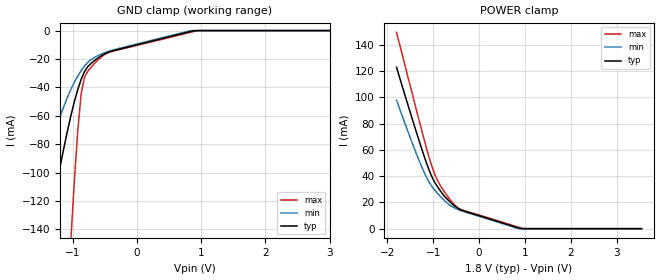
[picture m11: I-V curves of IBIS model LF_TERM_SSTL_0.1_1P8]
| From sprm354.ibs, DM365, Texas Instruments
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|   Model Cell LF_TERM_SSTL_0.1_1P8
|HALF_TERM_SSTL_0.1_1P8
[Model]   LF_TERM_SSTL_0.1_1P8
Model_type   Input
Polarity   Non-Inverting
Vinl =  0.8
Vinh =  1
C_comp   3.009089p   2.23501p   3.95018p
[Model Spec]
Vinl   0.8   0.75   0.85
Vinh   1   0.95   1.05
[Temperature Range]   25   125   -40
[Voltage Range]   1.8   1.7   1.9
[POWER_clamp]
|   voltage   I(typ)   I(min)   I(max)
-1.8V     123mA      97.85mA    149.6mA
-1.309V   67.13mA    52mA       82.68mA
-1.145V   49.92mA    39.06mA    61.14mA
-1.036V   40.14mA    32.51mA    48.14mA
-927.3mV  33.07mA    27.7mA     38.35mA
-818.2mV  27.54mA    23.61mA    31.37mA
-654.5mV  21.1mA     18.32mA    23.2mA
-490.9mV  16.23mA    15.02mA    16.68mA
-327.3mV  13.47mA    12.96mA    13.76mA
818.2mV   986.3uA    455.6uA    1.533mA
981.8mV   0A         0A         0A
3.545V    0A         0A         0A
[GND_clamp]
|   voltage   I(typ)   I(min)   I(max)
-1.8V     -238.9mA   -143.1mA   -823mA
-1.418V   -146.7mA   -89.2mA    -482.3mA
-1.364V   -133.7mA   -81.8mA    -433.5mA
-1.036V   -60.63mA   -41.79mA   -150.1mA
-981.8mV  -50.62mA   -36.69mA   -108.3mA
-927.3mV  -41.81mA   -32.19mA   -71.56mA
-872.7mV  -34.34mA   -28.23mA   -44.59mA
-818.2mV  -28.67mA   -24.82mA   -32.51mA
-654.5mV  -20.78mA   -18.67mA   -22.72mA
-436.4mV  -15.06mA   -14.43mA   -15.34mA
927.3mV   0A         0A         -167.4uA
3.545V    0A         0A         0A
